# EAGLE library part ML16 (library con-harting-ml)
HARTING
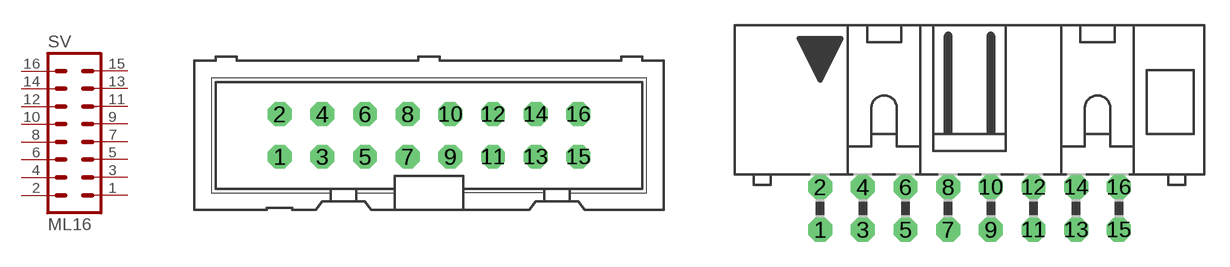
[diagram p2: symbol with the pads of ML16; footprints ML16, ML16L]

Designator prefix SV

## ML16 (OC_FARNELL: unknown; OC_NEWARK: unknown)  [ML16]
1  1  pas
2  2  pas
3  3  pas
4  4  pas
5  5  pas
6  6  pas
7  7  pas
8  8  pas
9  9  pas
10  10  pas
11  11  pas
12  12  pas
13  13  pas
14  14  pas
15  15  pas
16  16  pas

## ML16L (OC_FARNELL: unknown; OC_NEWARK: unknown)  [ML16L]
Pads as for ML16

## ML163M (OC_FARNELL: unknown; OC_NEWARK: unknown)  [3M_16]
Pads as for ML16

## ML163ML (OC_FARNELL: unknown; OC_NEWARK: unknown)  [3M_16L]
Pads as for ML16

## Footprint ML16 (pad centres in mm)
HARTING
drill 0.914 octagon: 1 -8.89,-1.27; 2 -8.89,1.27; 3 -6.35,-1.27; 4 -6.35,1.27; 5 -3.81,-1.27; 6 -3.81,1.27; 7 -1.27,-1.27; 8 -1.27,1.27; 9 1.27,-1.27; 10 1.27,1.27; 11 3.81,-1.27; 12 3.81,1.27; 13 6.35,-1.27; 14 6.35,1.27; 15 8.89,-1.27; 16 8.89,1.27

## Footprint ML16L (pad centres in mm)
HARTING
drill 0.914 octagon: 1 -8.89,-1.27; 2 -8.89,1.27; 3 -6.35,-1.27; 4 -6.35,1.27; 5 -3.81,-1.27; 6 -3.81,1.27; 7 -1.27,-1.27; 8 -1.27,1.27; 9 1.27,-1.27; 10 1.27,1.27; 11 3.81,-1.27; 12 3.81,1.27; 13 6.35,-1.27; 14 6.35,1.27; 15 8.89,-1.27; 16 8.89,1.27

## Footprint 3M_16 (pad centres in mm)
3M
drill 0.813 square: 1 -8.89,-1.27; 2 -8.89,1.27; 3 -6.35,-1.27; 4 -6.35,1.27; 5 -3.81,-1.27; 6 -3.81,1.27; 7 -1.27,-1.27; 8 -1.27,1.27; 9 1.27,-1.27; 10 1.27,1.27; 11 3.81,-1.27; 12 3.81,1.27; 13 6.35,-1.27; 14 6.35,1.27; 15 8.89,-1.27; 16 8.89,1.27

## Footprint 3M_16L (pad centres in mm)
3M
drill 0.813 square: 1 -8.89,-5.08; 2 -8.89,-2.54; 3 -6.35,-5.08; 4 -6.35,-2.54; 5 -3.81,-5.08; 6 -3.81,-2.54; 7 -1.27,-5.08; 8 -1.27,-2.54; 9 1.27,-5.08; 10 1.27,-2.54; 11 3.81,-5.08; 12 3.81,-2.54; 13 6.35,-5.08; 14 6.35,-2.54; 15 8.89,-5.08; 16 8.89,-2.54
hole 2.54 at -14.808,-3.277
hole 2.54 at 14.808,-3.277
